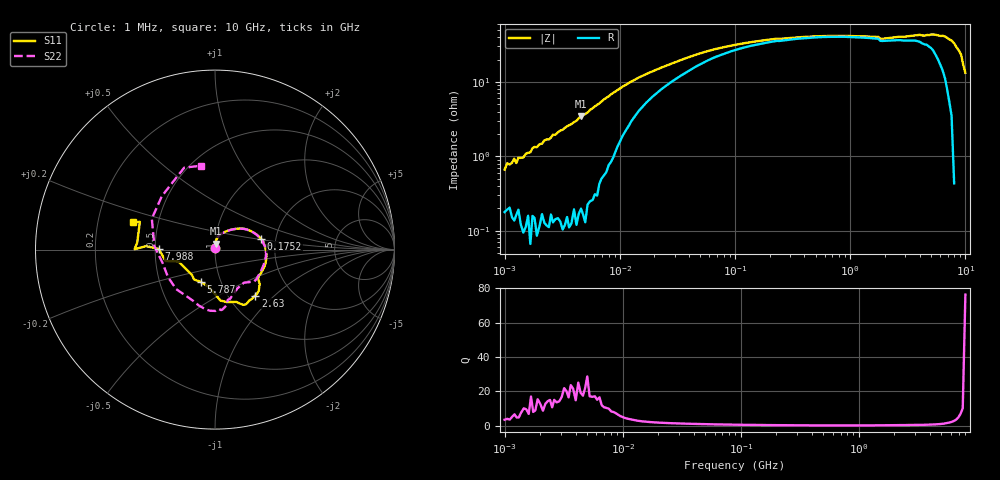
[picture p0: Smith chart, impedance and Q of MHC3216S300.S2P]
!Agilent Technologies,E5071C,MY46111244,A.11.31
!Date: Thu May 09 18:31:49 2019
!Data & Calibration Information:
!Freq	S11:SOLT2(ON)	S21:SOLT2(ON)	S12:SOLT2(ON)	S22:SOLT2(ON)
# Hz S dB R 50
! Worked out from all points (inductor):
!   201 points, 1 MHz to 10 GHz, reference 50 ohm
!   read as one part in series: L = 110 nH near 1.053 MHz
!   highest Q = 22 at 4.609 MHz (marker M1), where L = 120 nH
!   S11 on the Smith chart (normalised r, x): 1 MHz: 1.00, +0.01; 175.2 MHz: 1.67, +0.21; 2.63 GHz: 1.33, -0.77; 5.787 GHz: 0.80, -0.30; 7.988 GHz: 0.52, +0.00; 10 GHz: 0.36, +0.14
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1000000  -43.45 76.6  -0.01 -0.5  -0.03 -0.2  -43.40 85.7
1053043  -42.03 81.5  -0.02 -0.5  -0.02 -0.4  -42.35 80.5
1318257  -40.98 80.5  -0.02 -0.6  -0.03 -0.5  -39.90 83.6
1673262  -38.27 86.3  -0.00 -0.6  -0.01 -0.7  -39.33 84.8
4608546  -29.40 84.9  -0.03 -2.0  -0.02 -2.1  -29.48 85.9
4810209  -29.15 85.1  -0.02 -2.1  -0.02 -2.1  -29.23 85.7
1e7  -22.05 74.4  -0.16 -4.6  -0.17 -4.6  -22.04 74.4
2.206931e7  -17.19 52.4  -0.70 -7.1  -0.71 -7.2  -17.21 52.4
1.047129e8  -12.26 20.7  -2.16 -8.3  -2.17 -8.3  -12.25 20.5
1.75212e8  -11.57 13.1  -2.53 -7.9  -2.53 -7.9  -11.54 12.5
4.810209e8  -10.88 -2.0  -2.92 -8.8  -2.94 -8.8  -10.94 -3.1
1.59878e9  -10.92 -30.3  -3.03 -20.6  -3.06 -20.6  -10.92 -34.6
2.206931e9  -9.50 -43.3  -3.08 -28.4  -3.07 -28.4  -12.10 -57.7
2.630268e9  -9.36 -48.7  -3.24 -32.9  -3.24 -32.9  -11.67 -64.8
3.801894e9  -9.43 -64.2  -3.46 -44.4  -3.52 -44.5  -10.29 -77.8
4.83488e9  -10.90 -83.9  -3.42 -56.2  -3.45 -56.2  -9.59 -86.2
5.786901e9  -14.12 -114.0  -3.10 -69.1  -3.12 -69.1  -9.44 -98.9
6.661376e9  -14.28 -144.0  -2.73 -81.9  -2.72 -81.9  -10.35 -123.8
7.988146e9  -10.08 179.3  -2.30 -102.5  -2.30 -102.5  -9.41 176.7
8.792888e9  -6.97 179.7  -2.09 -116.2  -2.13 -116.1  -7.54 134.9
9.597629e9  -7.01 159.7  -2.12 -131.8  -2.11 -131.8  -6.24 110.6
1e10  -6.31 161.8  -1.86 -138.7  -1.85 -138.5  -6.49 99.6
